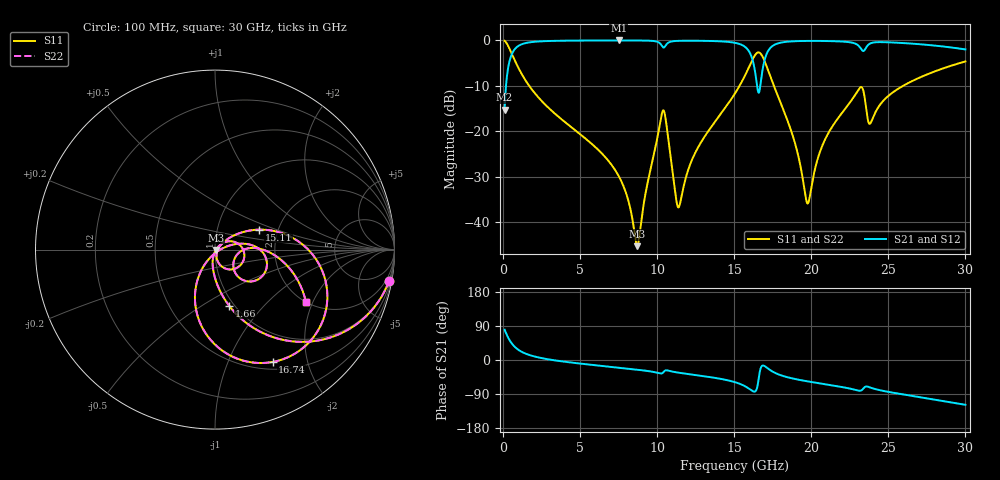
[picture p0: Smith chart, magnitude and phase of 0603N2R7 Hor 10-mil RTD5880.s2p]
# GHz S MA R 50
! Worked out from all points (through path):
!   3201 points, 100 MHz to 30 GHz, reference 50 ohm
!   highest |S21| = -0.04 dB at 7.5 GHz (marker M1); lowest = -15.3 dB at 100 MHz (marker M2)
!   group delay of S21, straight-line fit = 11.6 ps
!   lowest |S11| = -45.3 dB at 8.706 GHz (marker M3), VSWR 1.01, Z = 50.5 - j0.279 ohm
!   |S11| at or under -10 dB: 1.689 GHz to 15.35 GHz (13.66 GHz wide, 160 % of centre); 17.57 GHz to 25.97 GHz (8.403 GHz wide, 38.6 % of centre)
!   |S22| runs from -45.3 to -0.1 dB; largest |S21 - S12| = 0
!   S11 on the Smith chart (normalised r, x): 100 MHz: 1, -11; 1.66 GHz: 0.95, -0.66; 15.11 GHz: 1.59, +0.38; 16.74 GHz: 0.59, -1.47; 30 GHz: 2.00, -1.78
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0.1  0.9851 -10.2  0.1717 79.8  0.1717 79.8  0.9851 -10.2
0.5765313  0.7044 -46.9  0.7092 43.1  0.7092 43.1  0.7044 -46.9
1.660406  0.3213 -75.9  0.9456 13.8  0.9456 13.8  0.3213 -75.9
5.089563  0.08993 -98.2  0.9932 -9.9  0.9932 -9.9  0.08993 -98.2
7.50025  0.03204 -103.4  0.9956 -20.3  0.9956 -20.3  0.03204 -103.4
8.705594  0.005406 -30.7  0.9945 -25.5  0.9945 -25.5  0.005406 -30.7
10.06978  0.09492 29.5  0.9545 -34.4  0.9545 -34.4  0.09492 29.5
10.48091  0.158 -40.5  0.8446 -28.8  0.8446 -28.8  0.158 -40.5
11.40594  0.01457 -13.7  0.9861 -33.6  0.9861 -33.6  0.01457 -13.7
12.5085  0.05946 40.9  0.9885 -39.8  0.9885 -39.8  0.05946 40.9
15.05  0.26 25.2  0.9375 -58.5  0.9375 -58.5  0.26 25.2
15.10606  0.2693 24.4  0.9334 -59.2  0.9334 -59.2  0.2693 24.4
16.30206  0.6658 -20.2  0.5041 -83.5  0.5041 -83.5  0.6658 -20.2
16.74122  0.7034 -62.9  0.3659 -19.0  0.3659 -19.0  0.7034 -62.9
17.47003  0.351 -107.5  0.8623 -30.2  0.8623 -30.2  0.351 -107.5
19.69384  0.01681 -72.2  0.9836 -55.9  0.9836 -55.9  0.01681 -72.2
20.03956  0.02593 -4.2  0.9843 -58.3  0.9843 -58.3  0.02593 -4.2
20.93656  0.08361 15.7  0.9817 -64.2  0.9817 -64.2  0.08361 15.7
23.09497  0.292 -11.1  0.861 -81.0  0.861 -81.0  0.292 -11.1
23.80509  0.1205 -21.5  0.9192 -72.3  0.9192 -72.3  0.1205 -21.5
25.01978  0.2457 1.2  0.9499 -84.2  0.9499 -84.2  0.2457 1.2
30  0.5845 -30.0  0.7932 -118.2  0.7932 -118.2  0.5845 -30.0
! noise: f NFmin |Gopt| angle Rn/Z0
0.1  0.0003883  0.94  0.948  0.001444
3.417  0.003982  0.8077  10.31  0.004276
6.743  0.007032  0.7887  19.95  0.00665
10.06  0.02997  0.9213  29.45  0.07882
13.39  0.01779  0.8337  38.81  0.02012
16.7  0.2468  0.9841  48.11  2.949
20.03  0.0252  0.83  57.06  0.02417
23.35  0.1152  0.9545  65.75  0.4019
26.67  0.03055  0.8207  73.78  0.02297
30  0.03641  0.8329  81.72  0.02647
